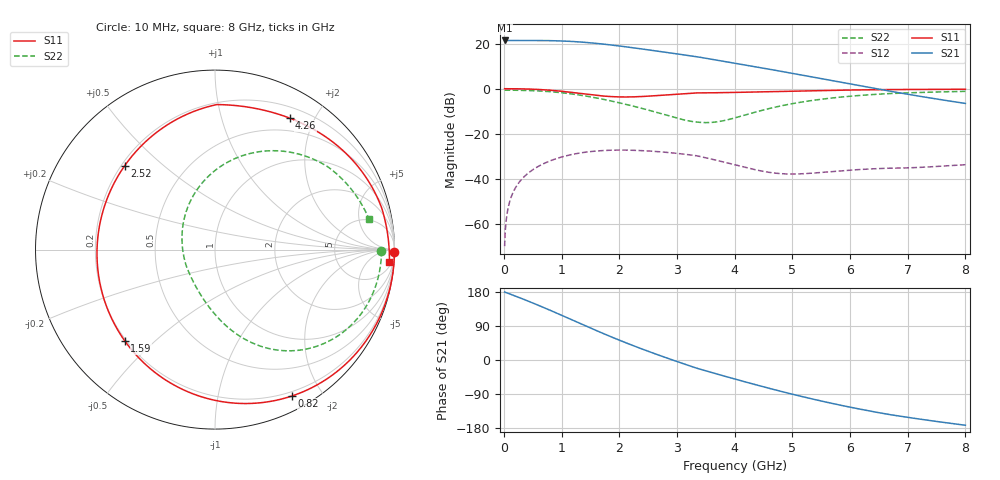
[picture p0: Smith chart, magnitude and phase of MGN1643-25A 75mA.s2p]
! Port[1] = GATE
! Port[2] = DRAIN
! [Type]  S-parameter s2p file touchstone ver. 1.0
! [Object]  MGN1643-25A
! [Bias]  75 mA
! [Version]  1.0
! [Date]  Tue May 19 13:03:48 2026
! [Source]  This file was created in JSC "ICC Milandr".
! [Disclaimer] Property of JSC "ICC Milandr". Unauthorized reproduction and/or distribution is strictly prohibited.
!  The file and the data are provided "AS IS" and with all faults and disclaim all warranties, express and implied, including
!  without limitation any implied warranties of merchantability, fitness for a particular purpose.
!  JSC "ICC Milandr" assumes no liability for:
!  1) the accuracy of the data provided;
!  2) the proper functioning of this data;
!  3) infringement of patents, copyrights or intellectual property rights resulting from the use of this data.
!  JSC "ICC Milandr" reserves the right to make changes to the products and the data without prior notice.
!  Please, be aware that your receipt and use of the file provided shall serve as acceptance of these terms and conditions.
!  If you do not accept these terms, you should return or destroy this file and any other accompanying information immediately.
# Hz S MA R 12.5
! freq  S11mag  S11ang  S21mag  S21ang  S12mag  S12ang  S22mag  S22ang
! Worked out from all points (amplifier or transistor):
!   800 points, 10 MHz to 8 GHz, reference 12.5 ohm
!   highest |S21| = 21.4 dB at 10 MHz (marker M1)
!   |S21| within 3 dB of that: start of sweep to 2.168 GHz
!   unconditionally stable (mu >= 1): 3.358 GHz to 7.245 GHz
!   at 1.34 GHz: K = 0.43, MSG = 24.5 dB, |S12| = -28.4 dB
!   at 4.01 GHz: K = 1.83, MAG = 17.2 dB, |S12| = -33.7 dB
!   at 8 GHz: K = 0.70, MSG = 13.6 dB, |S12| = -33.6 dB
!   S11 on the Smith chart (normalised r, x): 10 MHz: open; 820 MHz: 0.15, -1.64; 1.59 GHz: 0.19, -0.40; 2.52 GHz: 0.21, +0.38; 4.26 GHz: 0.33, +1.67; 8 GHz: 9, -25
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1e7  0.9998 -0.7  11.7 179.3  0.0003275 82.8  0.9276 -0.3
1.3e8  0.999 -9.3  11.68 172.6  0.004211 82.8  0.9266 -4.8
4.2e8  0.9839 -30.6  11.7 155.3  0.01358 67.8  0.9119 -15.8
6.2e8  0.9591 -46.0  11.67 142.8  0.01991 56.6  0.8896 -23.6
8.2e8  0.9213 -62.3  11.57 129.9  0.02591 45.0  0.8555 -31.6
1.09e9  0.8525 -85.9  11.26 111.9  0.03306 28.9  0.7906 -42.3
1.35e9  0.7773 -110.6  10.75 94.4  0.03839 13.2  0.711 -52.4
1.59e9  0.715 -134.8  10.11 78.4  0.0417 -1.1  0.6289 -61.3
1.82e9  0.6738 -158.5  9.408 63.5  0.04339 -14.3  0.5484 -69.4
2.04e9  0.6571 179.3  8.696 49.8  0.04382 -26.5  0.4743 -76.8
2.27e9  0.6622 157.7  7.957 36.1  0.04326 -38.6  0.4023 -84.7
2.52e9  0.6867 137.1  7.192 21.8  0.04175 -51.1  0.332 -94.2
2.68e9  0.7086 125.6  6.733 13.0  0.0404 -58.8  0.2916 -101.4
3.01e9  0.7591 105.5  5.871 -4.6  0.03694 -74.1  0.222 -121.4
3.33e9  0.8067 89.7  5.138 -21.1  0.03295 -88.3  0.1834 -151.5
3.65e9  0.8137 78.2  4.368 -35.2  0.0267 -94.2  0.182 175.8
4.01e9  0.8288 67.2  3.646 -50.6  0.02058 -96.5  0.2275 141.3
4.26e9  0.8423 60.5  3.214 -61.0  0.01718 -94.7  0.2802 122.9
4.79e9  0.8738 47.9  2.445 -82.3  0.01322 -81.2  0.4136 94.5
5.34e9  0.9047 36.6  1.823 -102.7  0.01352 -66.4  0.5491 73.1
6.67e9  0.9575 14.0  0.8921 -143.7  0.01742 -64.8  0.7797 36.3
8e9  0.974 -4.0  0.4722 -172.2  0.02082 -85.4  0.8751 11.1
